FUNCTION_BLOCK FileExample04_Configuration // any configuration of xbots and flyways - SetConfiguration, GetConfiguration. Configuration XML file 'PMCConfig.xml' must be on disc in the DemoFilesFolder.
VAR_INPUT
	Execute : BOOL;
	DemoFilesFolder : STRING(255);	//Folder that contains the PMCConfig.xml file
END_VAR
VAR_OUTPUT
	Done : BOOL;
END_VAR
VAR_IN_OUT
	PM_Controller : PMControllerType;	// the planar motor controller to use
END_VAR
VAR
	ReadFile : ReadFileOnDisk;
	send_config_array500000 : ARRAY[0..499999] OF SINT;
	read_config_array500000 : ARRAY[0..499999] OF SINT;
	PMC_DeactivateXbots1 : PMC_DeactivateXbots;
	PMC_SetConfiguration1 : PMC_Config_SetConfiguration;
	PMC_Reboot1 : PMC_Reboot;
	PMC_GetConfiguration1 : PMC_Config_GetConfiguration;	
END_VAR

// any configuration of xbots and flyways - SetConfiguration, GetConfiguration. Configuration XML file 'PMCConfig.xml' must be on disc in the DemoFilesFolder.

//read file from disk
ReadFile(Execute := Execute,file_path := CONCAT(STR1 := DemoFilesFolder,STR2 := '\PMCConfig.xml'),data := send_config_array500000);

//deactivate the PMC
PMC_DeactivateXbots1(Execute := ReadFile.Done,PM_Controller := PM_Controller);

//send the configuration to the PMC
PMC_SetConfiguration1(Execute := PMC_DeactivateXbots1.Done,nBytes := ReadFile.file_size,Bytes := send_config_array500000,PM_Controller := PM_Controller);

//reboot PMC to switch to the new configuration (restart PMT to update display in the GUI)
PMC_Reboot1(Execute := PMC_SetConfiguration1.Done,PM_Controller := PM_Controller);

//read the configuration from the PMC
PMC_GetConfiguration1(Execute := PMC_Reboot1.Done,Bytes := read_config_array500000,PM_Controller := PM_Controller);

Done := PMC_GetConfiguration1.Done;

END_FUNCTION_BLOCK
